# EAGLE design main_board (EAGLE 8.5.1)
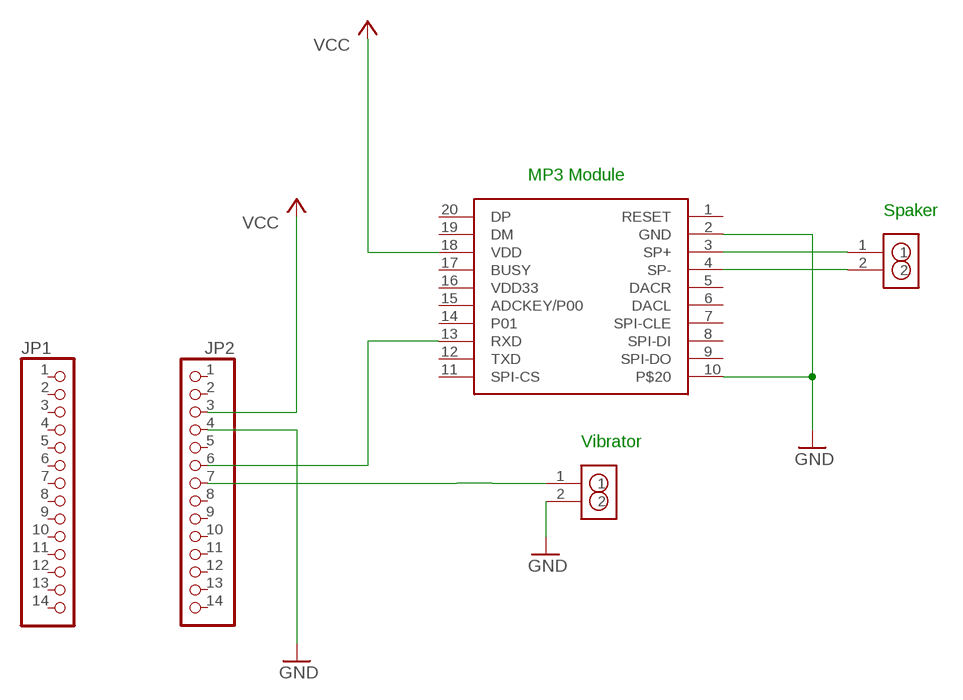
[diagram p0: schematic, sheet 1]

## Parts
JP1  PINHD-1X14-CB  [1X14-CB]
JP2  PINHD-1X14-CB  [1X14-CB]
U$1  VIBRATOR_PH  [PH]
U$2  MP3_MODULE  [WT2003B01_V3.XX]
U$3  VIBRATOR_PH  [PH]

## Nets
GND: JP2.4 U$1.2 U$2.2(GND) U$2.10
N$23: U$2.3(SP+) U$3.1
N$34: JP2.6 U$2.13(RXD)
N$35: JP2.7 U$1.1
N$37: U$2.4(SP-) U$3.2
VCC: JP2.3 U$2.18(VDD)
Unconnected: JP1.1 JP1.2 JP1.3 JP1.4 JP1.5 JP1.6 JP1.7 JP1.8 JP1.9 JP1.10 JP1.11 JP1.12 JP1.13 JP1.14 JP2.1 JP2.2 JP2.5 JP2.8 JP2.9 JP2.10 JP2.11 JP2.12 JP2.13 JP2.14 U$2.1(RESET) U$2.5(DACR) U$2.6(DACL) U$2.7(SPI-CLE) U$2.8(SPI-DI) U$2.9(SPI-DO) U$2.11(SPI-CS) U$2.12(TXD) U$2.14(P01) U$2.15(ADCKEY/P00) U$2.16(VDD33) U$2.17(BUSY) U$2.19(DM) U$2.20(DP)

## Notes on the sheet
- MP3 Module
- Spaker
- Vibrator

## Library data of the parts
JP1 JP2 = adafruit:PINHD-1X14: PIN HEADER
U$1 U$3 = custom_package:VIBRATOR_PH
U$2 = MP3_module:MP3_MODULE

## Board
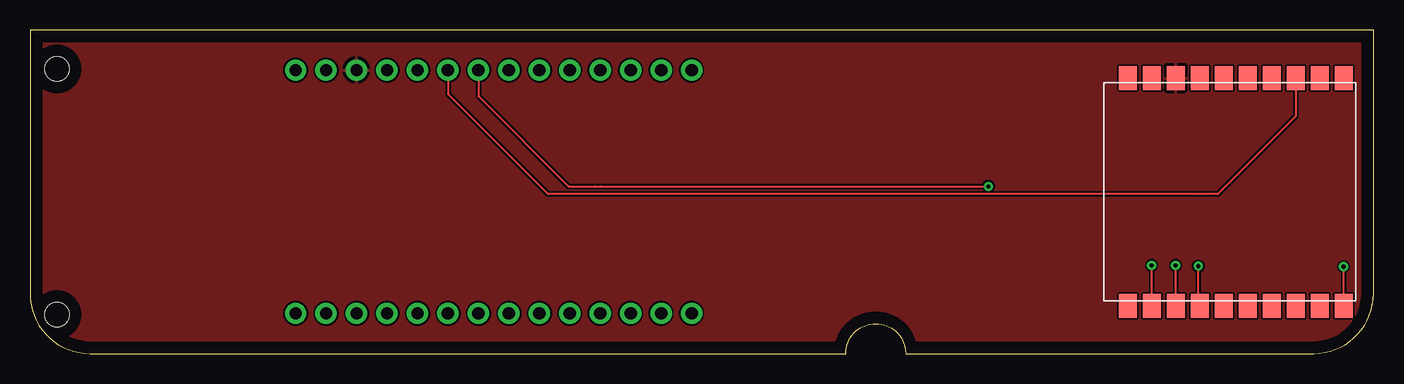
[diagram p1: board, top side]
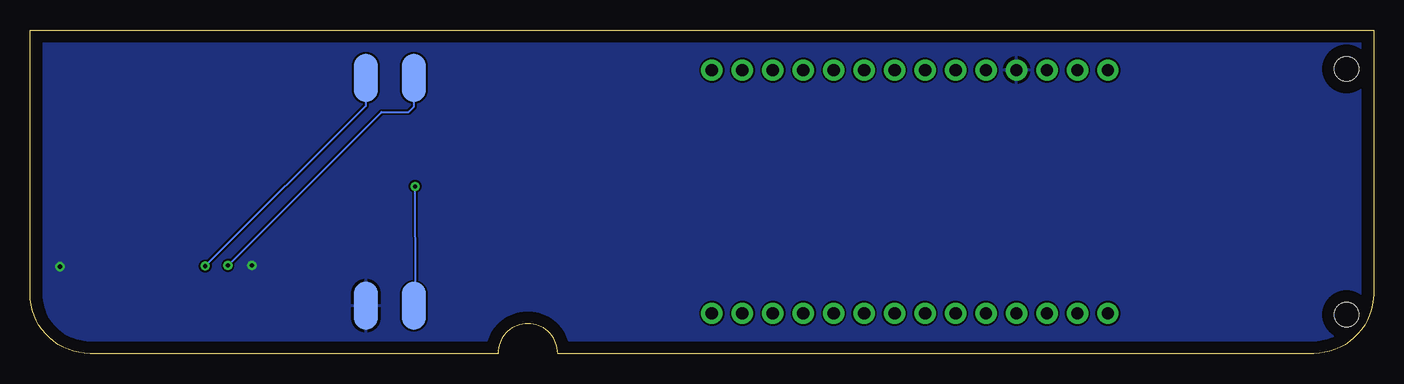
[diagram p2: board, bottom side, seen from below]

Size 112 x 27 mm. Coordinates in mm from the lower left corner, seen from the top.
Outline: 0,27 0,5 arc90 5,0 68,0 arc-90 70.5,2.5 arc-90 73,0 107,0 arc90 112,5 112,27 0,27
Copper layers (1*16): Top 0.035mm / dielectric 1.5mm / Bottom 0.035mm
Design rules "default": minimum track width 6mil, minimum drill 0.35mm, track to track 6mil, track to pad 6mil, pad to pad 6mil, via to via 6mil, smd to smd 6mil, copper to edge 40mil, drill to drill 6mil, minimum pad ring 10mil, minimum via ring 8mil, stop-mask expansion 4mil, vias tented up to drill 0mil, thermal gap 10mil
Holes 2 mm at 2.25,23.75 2.25,3.25

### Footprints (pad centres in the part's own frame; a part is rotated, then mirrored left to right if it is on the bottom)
1X14-CB = drill 1.016 pad 1.778: 1 -16.51,0; 2 -13.97,0; 3 -11.43,0; 4 -8.89,0; 5 -6.35,0; 6 -3.81,0; 7 -1.27,0; 8 1.27,0; 9 3.81,0; 10 6.35,0; 11 8.89,0; 12 11.43,0; 13 13.97,0; 14 16.51,0
PH = smd 2 x 4: 1 -2,0; 2 2,0
WT2003B01_V3.XX = smd 2 x 1.5: 1 -9.5,8.5; 2 -9.5,6.5; 3 -9.5,4.5; 4 -9.5,2.5; 5 -9.5,0.5; 6 -9.5,-1.5; 7 -9.5,-3.5; 8 -9.5,-5.5; 9 -9.5,-7.5; 10 -9.5,-9.5; 11 9.5,-9.5; 12 9.5,-7.5; 13 9.5,-5.5; 14 9.5,-3.5; 15 9.5,-1.5; 16 9.5,0.5; 17 9.5,2.5; 18 9.5,4.5; 19 9.5,6.5; 20 9.5,8.5

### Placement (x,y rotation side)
JP1  38.65,3.35 0 top
JP2  38.65,23.65 0 top
U$1  82,3.98 180 bottom
U$2  100,13.5 90 top
U$3  82,23 180 bottom

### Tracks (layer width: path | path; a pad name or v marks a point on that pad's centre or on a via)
GND  (via drill 0.35)
  Top 0.152: U$2.10 v109.5,7.25 | U$2.2 v93.5,7.35
  pour Bottom: -1,28 -1,3 arc90 4,-2 108,-2 arc90 113,3 113,26 111,28
N$23  (via drill 0.35)
  Top 0.152: U$2.3 v95.5,7.35
  Bottom 0.152: v95.5,7.35 82.7,20.15 80.45,20.15 80,20.6 U$3.1
N$34
  Top 0.152: 34.9,23.62 JP2.6 34.84,21.66 43.2,13.3 97.35,13.3 97.85,13.3 99,13.3 105.5,19.8 U$2.13
N$35  (via drill 0.35)
  Top 0.152: v79.9,13.95 47.6,13.95 47.08,13.95 44.9,13.95 37.38,21.47 JP2.7
  Bottom 0.152: v79.9,13.95 79.86,5.49 79.86,4.12 U$1.1
N$37  (via drill 0.35)
  Top 0.152: U$2.4 97.4,4.1 v97.4,7.3
  Bottom 0.152: v97.4,7.3 84,20.7 U$3.2
VCC
  pour Top: -0.8,27.35 -0.8,-0.1 -0.5,-0.4 112.35,-0.4 112.7,-0.05 112.7,26.65 111.85,27.5 -0.65,27.5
